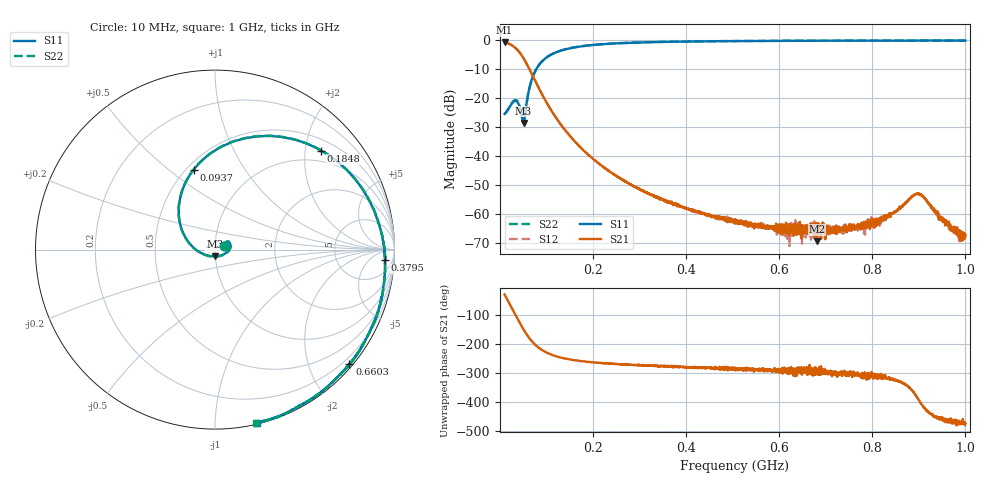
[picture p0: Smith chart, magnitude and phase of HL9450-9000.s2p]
! 7/10/2020 11:13:37 AM
! H:\PRODUCTION_DATA\9450\10006\HL9450_10006_38P9M_.S2P
! CHANNEL.1
! TR.MEASUREMENT
! CORRECTED.DATA
# GHZ S RI R 50.0
! FREQ.GHZ  S11RE  S11IM  S21RE  S21IM  S12RE  S12IM  S22RE  S22IM
!; PortSelection: Port_12
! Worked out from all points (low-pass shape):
!   2000 points, 10 MHz to 1 GHz, reference 50 ohm
!   highest |S21| = -0.63 dB at 10 MHz (marker M1); lowest = -69.3 dB at 681.1 MHz (marker M2)
!   |S21| within 3 dB of the highest: start of sweep to 39.45 MHz
!   lowest |S11| = -28.4 dB at 50.61 MHz (marker M3), VSWR 1.08, Z = 49.7 - j3.76 ohm
!   |S11| at or under -10 dB: start of sweep to 77.8 MHz
!   |S22| runs from -28.1 to 0.0 dB; largest |S21 - S12| = 0.0014
!   S11 on the Smith chart (normalised r, x): 10 MHz: 1.11, +0.04; 93.7 MHz: 0.54, +0.61; 184.8 MHz: 0.74, +2.34; 379.5 MHz: 16, -19; 660.3 MHz: 0.07, -2.71; 1 GHz: 0.01, -1.27
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0.01  0.0507 0.0187  0.8063 -0.4631  0.8076 -0.4637  0.0501 0.0186
0.0204002  0.059 0.0382  0.4217 -0.7596  0.4217 -0.7599  0.058 0.0398
0.02832416  0.0752 0.0423  0.0722 -0.7923  0.0724 -0.7932  0.0759 0.0454
0.03971486  0.0805 0.00279  -0.3169 -0.5727  -0.3175 -0.5725  0.0847 0.0049
0.05061031  -0.00126 -0.0378  -0.4271 -0.2455  -0.4273 -0.2457  0.00326 -0.0393
0.06942972  -0.1881 0.1207  -0.2473 0.0551  -0.2476 0.0549  -0.1881 0.1179
0.09369685  -0.1197 0.4443  -0.0748 0.0735  -0.0749 0.0734  -0.1205 0.4454
0.1273737  0.1894 0.6244  -0.0157 0.0352  -0.0158 0.0352  0.1914 0.6262
0.1754127  0.5415 0.5764  -0.00245 0.0135  -0.00252 0.0135  0.5445 0.5778
0.1848224  0.5909 0.5509  -0.00173 0.0114  -0.00175 0.0115  0.5946 0.5512
0.2521761  0.8252 0.3317  -4.53e-05 0.00447  -1.48e-05 0.00448  0.8287 0.3289
0.3403302  0.9353 0.0514  0.000256 0.00184  0.000183 0.00195  0.9378 0.0477
0.3794547  0.9468 -0.0588  0.000221 0.00146  0.000244 0.00145  0.9485 -0.0645
0.5052476  0.9029 -0.3609  0.00019 0.000734  0.000188 0.000737  0.9016 -0.3655
0.6602601  0.7487 -0.6392  0.000224 0.000394  0.000367 0.000546  0.7452 -0.6483
0.6701651  0.7378 -0.653  0.000314 0.00045  0.000492 0.000517  0.7325 -0.6598
0.6810605  0.7225 -0.6696  0.000151 0.000309  0.000162 0.000481  0.7184 -0.6763
0.7766433  0.5909 -0.7941  0.000348 0.000433  0.000375 0.000484  0.585 -0.7983
0.8350825  0.5037 -0.8516  0.000717 0.000624  0.000705 0.000617  0.4966 -0.8568
0.9004552  0.4002 -0.9078  0.00184 -0.00127  0.00178 -0.00127  0.3933 -0.9134
0.9697899  0.2861 -0.9514  -0.000204 -0.000479  -0.000188 -0.000492  0.2785 -0.9535
1  0.2356 -0.9641  -0.000169 -0.000379  -0.000178 -0.000336  0.2262 -0.9656
